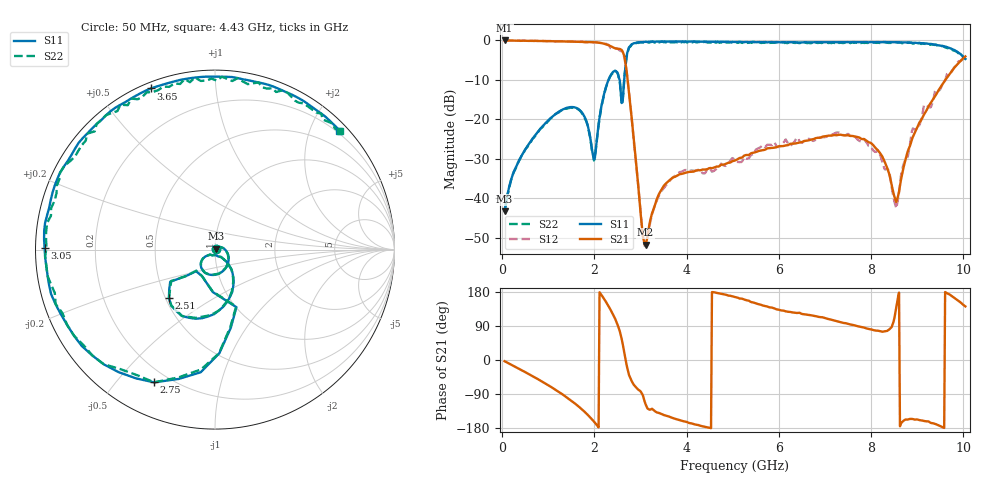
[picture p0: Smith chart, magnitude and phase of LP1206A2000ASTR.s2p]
!Instrument:	"HEWLETT PACKARD,8720ES,US39172150,7.62 "
!	LP1206	High	Performance	Low	Pass	Filters
!	P/N	LP1206A2000ASTR	6	May	2019
#	MHz	S	dB	R	50
!	Frq	S11(dB)	S11(deg)	S21(dB)	S21(deg)	S12(dB)	S12(deg)	S22(dB)	S22(deg)
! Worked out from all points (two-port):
!   501 points, 50 MHz to 10.05 GHz, reference 50 ohm
!   highest |S21| = -0.04 dB at 50 MHz (marker M1); lowest = -51.8 dB at 3.11 GHz (marker M2)
!   |S21| within 3 dB of the highest: start of sweep to 2.618 GHz
!   lowest |S11| = -43.3 dB at 50 MHz (marker M3), VSWR 1.01, Z = 50.5 + j0.496 ohm
!   |S11| at or under -10 dB: start of sweep to 2.306 GHz; 2.544 GHz to 2.646 GHz (101.8 MHz wide, 3.92 % of centre)
!   |S22| runs from -43.4 to -0.3 dB; largest |S21 - S12| = 0.051
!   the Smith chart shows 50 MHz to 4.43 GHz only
!   S11 on the Smith chart (normalised r, x): 50 MHz: 1.01, +0.01; 2.51 GHz: 0.52, -0.33; 2.75 GHz: 0.14, -0.63; 3.05 GHz: 0.03, +0.01; 3.65 GHz: 0.03, +0.68; 4.43 GHz: 0.15, +2.48
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50  -43.31 46.0  -0.04 -3.2  -0.05 -3.3  -43.41 45.8
1050  -19.71 -44.8  -0.21 -70.5  -0.16 -70.9  -19.81 -44.8
1730  -18.34 -130.5  -0.39 -130.4  -0.40 -130.7  -18.54 -130.6
1990  -30.25 -96.7  -0.48 -162.6  -0.48 -163.0  -30.45 -96.7
2250  -11.82 -68.2  -1.02 153.3  -0.86 155.4  -11.92 -68.4
2510  -8.55 -133.4  -2.15 90.3  -2.19 88.6  -8.55 -133.4
2630  -12.51 -93.0  -3.42 31.0  -3.73 29.4  -12.61 -93.1
2750  -1.79 -114.7  -13.28 -39.6  -13.00 -42.2  -1.79 -114.7
3050  -0.45 179.3  -49.56 -93.0  -49.65 -96.3  -0.55 179.3
3110  -0.37 171.2  -51.84 -116.9  -52.18 -115.9  -0.47 171.0
3390  -0.34 137.8  -39.21 -139.4  -39.54 -138.5  -0.34 137.8
3650  -0.30 111.7  -35.25 -150.9  -35.38 -154.2  -0.50 111.5
4430  -0.36 43.7  -32.69 -177.4  -33.06 -174.2  -0.36 43.5
5050  -0.40 -6.2  -30.47 166.0  -30.68 165.2  -0.60 -6.2
5950  -0.44 -79.7  -27.10 133.8  -26.84 131.8  -0.54 -79.9
6730  -0.50 -144.5  -25.08 117.4  -25.41 117.1  -0.50 -144.7
7470  -0.47 154.1  -24.08 96.5  -23.91 97.3  -0.67 154.1
8390  -0.48 77.4  -33.62 80.0  -33.12 87.0  -0.68 77.4
8550  -0.47 63.8  -41.00 138.4  -42.61 145.0  -0.47 63.7
8910  -0.65 31.8  -24.49 -155.9  -22.31 -153.5  -0.85 31.6
9250  -0.89 -0.3  -16.72 -162.1  -16.92 -171.0  -1.09 -0.3
10050  -4.72 -92.3  -4.07 141.5  -3.71 140.9  -4.82 -92.4
